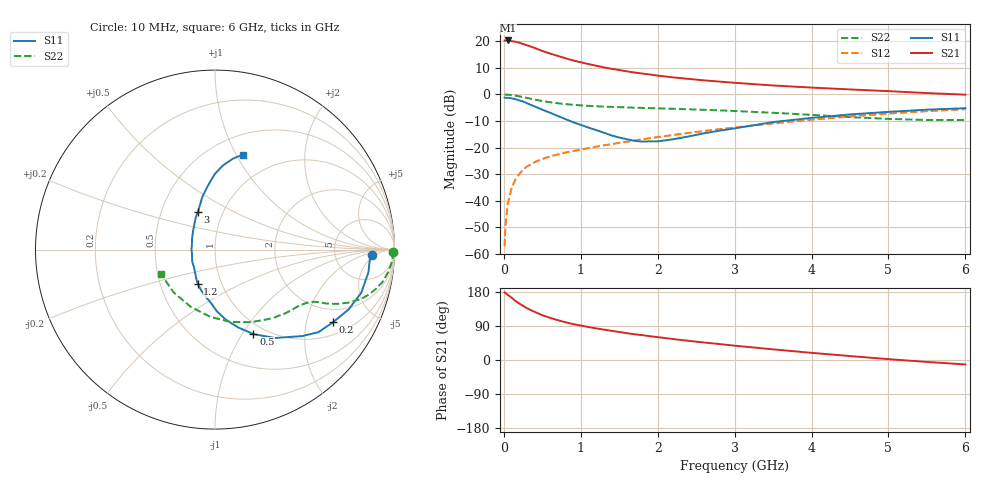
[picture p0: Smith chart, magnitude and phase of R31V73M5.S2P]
! SIEMENS Small Signal Semiconductors
! BFR181
! Si NPN RF Bipolar Junction Transistor in SOT23
! VCE = 1.75 V  IC = 3.5 mA
! Common Emitter S-Parameters:  May  1996
# GHz  S  MA  R  50
!  f  S11  S21  S12  S22
! GHz  MAG  ANG  MAG  ANG  MAG  ANG  MAG  ANG
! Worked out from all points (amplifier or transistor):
!   36 points, 10 MHz to 6 GHz, reference 50 ohm
!   highest |S21| = 20.3 dB at 50 MHz (marker M1)
!   |S21| within 3 dB of that: start of sweep to 417.4 MHz
!   unconditionally stable (mu >= 1): 1.252 GHz to 3.144 GHz
!   at 250 MHz: K = 0.34, MSG = 23.6 dB, |S12| = -28.3 dB
!   at 1.4 GHz: K = 1.04, MAG = 13.0 dB, |S12| = -18.7 dB
!   at 6 GHz: K = 0.86, MSG = 2.7 dB, |S12| = -5.5 dB
!   S11 on the Smith chart (normalised r, x): 10 MHz: 14, -3; 200 MHz: 1.44, -2.88; 500 MHz: 0.87, -1.12; 1.2 GHz: 0.77, -0.31; 3 GHz: 0.76, +0.34; 6 GHz: 0.70, +1.07
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0.01  0.8755 -1.8  10.26 178.5  0.0014 86.4  0.9939 -0.7
0.02  0.8646 -3.3  10.22 176.6  0.0032 87.6  0.9924 -1.6
0.05  0.8642 -8.5  10.36 172.0  0.0087 85.2  0.9883 -3.9
0.1  0.8494 -16.5  10.06 164.5  0.0173 81.9  0.9728 -7.5
0.15  0.8152 -24.2  9.81 156.0  0.025 76.7  0.9501 -11.0
0.2  0.7724 -31.6  9.425 149.2  0.0317 73.9  0.9212 -13.9
0.3  0.6838 -44.8  8.422 136.7  0.044 68.0  0.8614 -18.5
0.4  0.5949 -55.9  7.505 127.0  0.0533 63.7  0.802 -21.6
0.5  0.5171 -65.5  6.577 118.1  0.0608 61.4  0.7507 -23.7
0.6  0.4535 -73.3  5.892 111.4  0.0684 59.8  0.7151 -25.0
0.7  0.3947 -81.3  5.312 105.1  0.0742 59.2  0.6831 -26.0
0.8  0.3438 -88.3  4.797 99.7  0.0806 58.8  0.6584 -26.6
0.9  0.3012 -93.8  4.366 94.8  0.0862 59.0  0.6378 -27.2
1.1  0.2379 -109.2  3.733 87.1  0.098 59.4  0.6096 -28.6
1.2  0.2133 -116.9  3.469 83.4  0.1041 59.7  0.5994 -29.4
1.6  0.1439 -151.7  2.715 70.7  0.1294 60.3  0.5701 -32.8
2.2  0.1434 152.8  2.092 55.3  0.1727 60.1  0.5375 -39.8
3  0.2301 114.4  1.656 37.8  0.2391 56.7  0.488 -52.5
3.5  0.3021 103.5  1.474 28.1  0.285 53.1  0.4519 -63.4
4.5  0.4207 90.2  1.242 10.4  0.3859 43.2  0.3755 -94.1
5.5  0.517 78.8  1.061 -5.1  0.4848 30.5  0.3315 -134.0
6  0.5517 73.6  0.99 -11.8  0.5295 23.3  0.3306 -155.6
